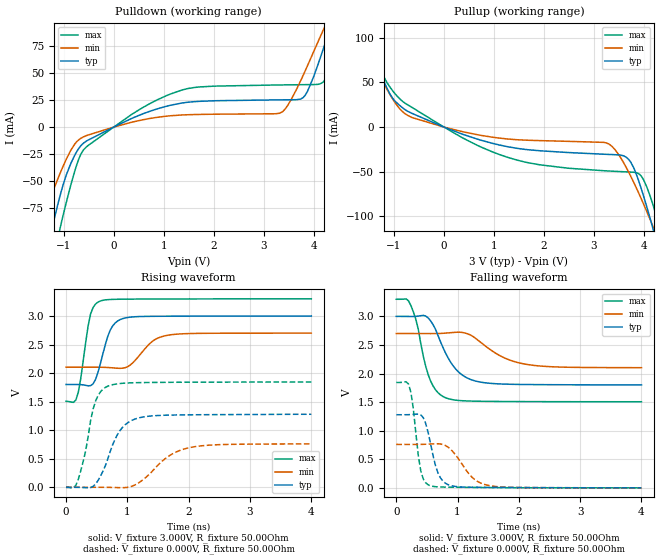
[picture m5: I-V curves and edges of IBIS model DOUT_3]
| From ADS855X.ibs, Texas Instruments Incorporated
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|   Output 3.0V Model
[Model]   DOUT_3
Model_type   Output
|Signals   BUSY/INT
Vmeas = 1.523V
Cref = 30.00pF
| C_comp   obtained at 36MHz
| variable   typ   min   max
|C_comp Output Low
C_comp   4.178pF   3.202pF   5.099pF
|C_comp Output High
|C_comp   4.247pF   3.275pF   5.243pF
[Model Spec]
Vmeas   1.52V   1.34V   1.77V
Vref   2.50V   0.50V   3.00V
|Junction Temperature
[Temperature Range]   40.0   125.0   -40.0
[Voltage range]   3.0V   2.70V   3.3V
[Pullup reference]   3.0V   2.7V   3.3V
[power clamp reference]   3.0V   2.7V   3.3V
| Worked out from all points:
|   slope of the pulldown table from 0 to 0.45 V, typ, clamps not added: 46.1 ohm
|   slope of the pullup table from 0 to 0.45 V, typ, clamps not added: 47.6 ohm
|   falling waveform, V_fixture 3.000V, R_fixture 50.00Ohm: 20-80 % time 359ps typ, 552ps min, 242ps max; typ from 3 V to 1.8 V
|   rising waveform, V_fixture 3.000V, R_fixture 50.00Ohm: 20-80 % time 197ps typ, 315ps min, 149ps max; typ from 1.8 V to 3 V
|   rising waveform, V_fixture 0.000V, R_fixture 50.00Ohm: 20-80 % time 312ps typ, 499ps min, 212ps max; typ from 0 V to 1.28 V
|   falling waveform, V_fixture 0.000V, R_fixture 50.00Ohm: 20-80 % time 176ps typ, 329ps min, 124ps max; typ from 1.28 V to 0 V
[Pulldown]
|   Voltage   I(typ)   I(min)   I(max)
-3V       -493.5mA   -328.7mA   -702.6mA
-1.482V   -144.9mA   -93.75mA   -210.6mA
-1.222V   -91.05mA   -60.13mA   -130.9mA
-1.074V   -63.32mA   -42.73mA   -93.54mA
-627.4mV  -15.75mA   -9.559mA   -22.54mA
576.4mV   12.15mA    6.695mA    17.93mA
1.473V    22.93mA    11.39mA    35.55mA
3.321V    25.18mA    12.81mA    38.97mA
3.834V    29.57mA    52.23mA    39.24mA
4.231V    77.55mA    93.58mA    44.03mA
4.626V    130.9mA    131.1mA    111.8mA
5.999V    252.7mA    219.9mA    290mA
[Pullup]
|   Voltage   I(typ)   I(min)   I(max)
-3V       226.4mA    192.1mA    270.6mA
-1.885V   136.6mA    115.4mA    166.2mA
-1.55V    96.55mA    83.71mA    114.7mA
-1.175V   47.75mA    45.61mA    53.31mA
-639.8mV  15.32mA    10.68mA    22mA
1.267V    -21.91mA   -13.31mA   -33.75mA
3.309V    -30.66mA   -19.21mA   -49.22mA
3.74V     -39.35mA   -55.1mA    -50.41mA
3.962V    -71.05mA   -81.77mA   -55.79mA
4.175V    -111.8mA   -110mA     -85.27mA
4.301V    -137.8mA   -127.6mA   -113.4mA
5.999V    -527.8mA   -397.6mA   -658.4mA
[Ramp]
R_load = 50.00Ohm
|   typ   min   max
dV/dt_r   767.588mV/312.304ps 456.037mV/498.579ps   1.106V/212.465ps
dV/dt_f   719.581mV/358.502ps 358.322mV/552.147ps   1.076V/241.501ps
[Falling Waveform]
V_fixture = 3.000V
V_fixture_min = 2.700V
V_fixture_max = 3.300V
R_fixture = 50.00Ohm
|   Time   V(typ)   V(min)   V(max)
0s        3V         2.7V       3.3V
240ps     2.999V     2.7V       3.187V
320ps     3.001V     2.7V       2.944V
520ps     2.973V     2.699V     1.983V
640ps     2.774V     2.7V       1.716V
800ps     2.367V     2.708V     1.578V
1.04ns    2.005V     2.723V     1.527V
1.4ns     1.846V     2.527V     1.515V
2.16ns    1.808V     2.155V     1.509V
4ns       1.801V     2.103V     1.507V
[Rising Waveform]
V_fixture = 3.000V
V_fixture_min = 2.700V
V_fixture_max = 3.300V
R_fixture = 50.00Ohm
|   Time   V(typ)   V(min)   V(max)
0s        1.801V     2.103V     1.507V
160ps     1.801V     2.103V     1.53V
240ps     1.798V     2.103V     1.91V
400ps     1.78V      2.103V     3.037V
560ps     2.169V     2.103V     3.263V
720ps     2.753V     2.095V     3.289V
960ps     2.965V     2.093V     3.295V
1.4ns     2.994V     2.55V      3.297V
1.64ns    2.996V     2.659V     3.298V
4ns       3V         2.7V       3.3V
[Rising Waveform]
V_fixture = 0.000V
V_fixture_min = 0.000V
V_fixture_max = 0.000V
R_fixture = 50.00Ohm
|   Time   V(typ)   V(min)   V(max)
0s        -885.7nV   -1.489uV   -525.3nV
160ps     405.1uV    12.3uV     36.11mV
320ps     -6.546mV   181.8uV    640.3mV
480ps     56.17mV    451.2uV    1.507V
680ps     495.9mV    -767.9uV   1.771V
880ps     994.4mV    -6.557mV   1.817V
1.2ns     1.219V     89.63mV    1.833V
1.64ns    1.263V     520.4mV    1.838V
2ns       1.269V     691.1mV    1.84V
4ns       1.279V     760.1mV    1.844V
[Falling Waveform]
V_fixture = 0.000V
V_fixture_min = 0.000V
V_fixture_max = 0.000V
R_fixture = 50.00Ohm
|   Time   V(typ)   V(min)   V(max)
0s        1.279V     760.1mV    1.844V
200ps     1.28V      759.7mV    1.815V
280ps     1.285V     759.7mV    1.364V
400ps     1.276V     760.7mV    294.1mV
520ps     967.7mV    764.8mV    52.82mV
680ps     261mV      770.9mV    16.79mV
880ps     42.01mV    681mV      11.34mV
1.24ns    10.39mV    180.9mV    7.385mV
1.52ns    7.799mV    38.94mV    4.655mV
4ns       -885.7nV   -1.489uV   -525.3nV
